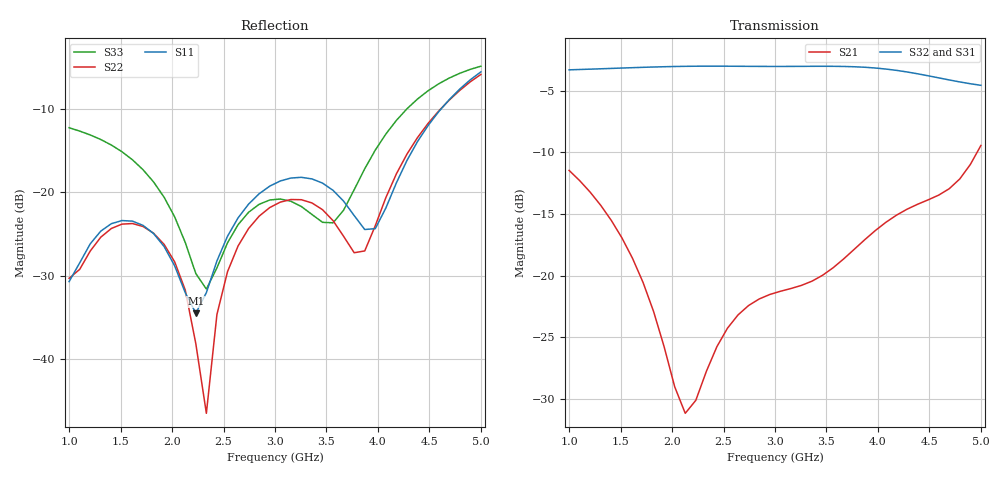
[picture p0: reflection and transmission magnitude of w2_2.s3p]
# GHZ S RI R 50
!Output file by EM3DS 5.12 Built 2
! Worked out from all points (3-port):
!   40 points, 1 GHz to 5 GHz, reference 50 ohm
!   strongest paths, dB at 1 GHz, 2.026 GHz, 3.051 GHz, 4.077 GHz, 5 GHz:
!     S32: -3.3, -3.0, -3.0, -3.2, -4.6
!     S31: -3.3, -3.0, -3.1, -3.3, -5.0
!     S21: -11.5, -29.0, -21.3, -15.7, -9.4
!   lowest |S11| = -34.5 dB at 2.231 GHz (marker M1), VSWR 1.04, Z = 48.6 + j1.27 ohm
!   |S11| at or under -10 dB: start of sweep to 4.615 GHz
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1  -0.0073 0.0282  -0.1303 -0.2331  -0.0794 -0.6833
   -0.1303 -0.2331  0.00271 0.0304  -0.0819 -0.6785
   -0.0794 -0.6833  -0.0819 -0.6785  -0.0811 0.2296
1.717949  -0.0194 0.0602  -0.0892 0.029  -0.6599 -0.2346
          -0.0892 0.029  -0.0067 0.0619  -0.6606 -0.2304
          -0.6599 -0.2346  -0.6606 -0.2304  0.0236 0.1343
2.230769  -0.0136 0.013  0.0304 0.00695  -0.622 0.3315
          0.0304 0.00695  0.00521 0.0112  -0.621 0.3378
          -0.622 0.3315  -0.621 0.3378  0.00155 0.0325
2.333333  -0.0246 0.00445  0.0393 -0.0111  -0.5576 0.4307
          0.0393 -0.0111  -0.00461 0.00106  -0.5557 0.4375
          -0.5576 0.4307  -0.5557 0.4375  -0.0141 0.0222
2.538462  -0.0544 7.97e-05  0.0403 -0.046  -0.3833 0.5895
          0.0403 -0.046  -0.0325 -0.00738  -0.3788 0.5969
          -0.3833 0.5895  -0.3788 0.5969  -0.0462 0.0183
3.051282  -0.0965 0.0657  -0.000742 -0.0863  0.1844 0.6746
          -0.000742 -0.0863  -0.0753 0.0439  0.1975 0.6773
          0.1844 0.6746  0.1975 0.6773  -0.0556 0.0721
3.564103  -0.034 0.0968  -0.03 -0.1032  0.6323 0.3003
          -0.03 -0.1032  -0.0284 0.0613  0.645 0.2878
          0.6323 0.3003  0.645 0.2878  0.0597 0.027
3.871795  -0.0301 0.0516  -0.0659 -0.1232  0.6921 -0.0631
          -0.0659 -0.1232  -0.0405 0.0183  0.6953 -0.0817
          0.6921 -0.0631  0.6953 -0.0817  0.0793 -0.1132
4.487179  -0.2052 0.1446  -0.1829 -0.0874  0.251 -0.5886
          -0.1829 -0.0874  -0.2171 0.1404  0.2415 -0.5997
          0.251 -0.5886  0.2415 -0.5997  -0.25 -0.3195
5  0.0456 0.5245  -0.3356 -0.0298  -0.2305 -0.5151
   -0.3356 -0.0298  0.06 0.5047  -0.2555 -0.5333
   -0.2305 -0.5151  -0.2555 -0.5333  -0.5625 -0.0895
